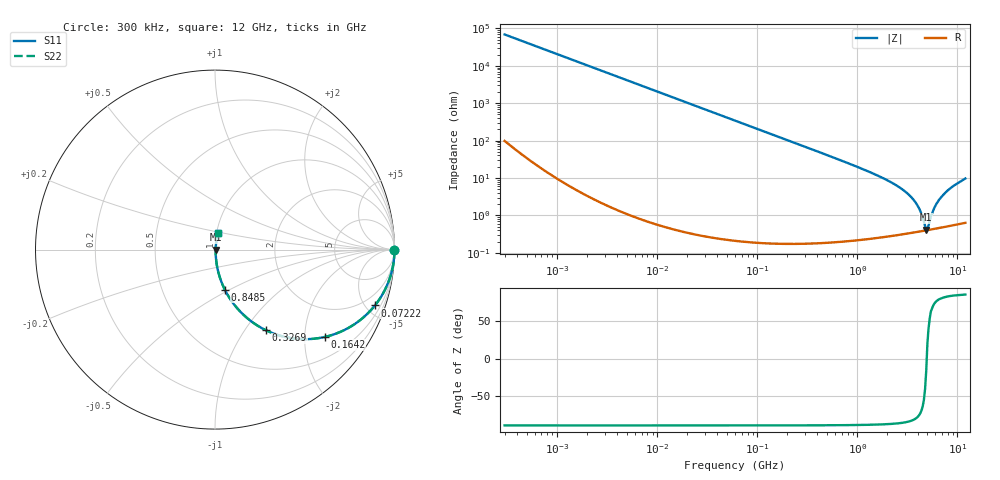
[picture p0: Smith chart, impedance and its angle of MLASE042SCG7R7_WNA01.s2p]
! MLASE042SCG7R7_WNA01  S-PARAMETER MODEL  ( General Type )
! Model Generated by TAIYO YUDEN Corporation (http://www.ty-top.com)
! Version 1.0
! TAIYO YUDEN Control No. 130801
! Copyright(c) 2013 TAIYO YUDEN CO.,LTD. All Rights Reserved.
! Product Description (link to TY-COMPAS)
! https://ds.yuden.co.jp/TYCOMPAS/or/detail?pn=MLASE042SCG7R7BWNA01&u=M
! Products Name : Multilayer Ceramic Capacitors
! Characteristics :
!  Capacitance : 7.7 pF , Rated Voltage : 16V , TCC : CG / C0G
!  Case Size : 0.4 x 0.2 / 0.016 x 0.008 [mm/inch] , Thickness : 0.2 / 0.008 [mm/inch]
!  (Conditions: Temperature = 25 degC , DC Bias Current/Voltage = 0A / 0V)
! External Node Assignments :
!  1  o---| |---o  2
! GND o---------o GND
! Frequency Range : 0.3MHz  -  12000MHz  [ 401 STEP ]
# MHz S RI R 50
! Freq[MHz].  S11 Real  S11 Imag  S21 Real  S21 Imag  S12 Real  S12 Imag  S22 Real  S22 Imag
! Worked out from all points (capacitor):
!   401 points, 300 kHz to 12 GHz, reference 50 ohm
!   read as one part in series: C = 7.7 pF near 316.3 kHz
!   lowest |Z| = 415 mohm at 4.875 GHz (marker M1)
!   series resonance near 4.934 GHz, so ESL is about 140 pH
!   S11 on the Smith chart (normalised r, x): 300 kHz: open; 72.22 MHz: 1.00, -5.72; 164.2 MHz: 1.00, -2.52; 326.9 MHz: 1.00, -1.26; 848.5 MHz: 1.00, -0.47; 12 GHz: 1.01, +0.19
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0.3  1 -0.00145  4.17e-06 0.00145  4.17e-06 0.00145  1 -0.00145
1.769972  0.9999 -0.00856  7.62e-05 0.00856  7.62e-05 0.00856  0.9999 -0.00856
10.44266  0.9974 -0.0504  0.00256 0.0504  0.00256 0.0504  0.9974 -0.0504
27.10171  0.9831 -0.1289  0.0169 0.1289  0.0169 0.1289  0.9831 -0.1289
60  0.9221 -0.2676  0.0779 0.2676  0.0779 0.2676  0.9221 -0.2676
72.22496  0.891 -0.3113  0.109 0.3113  0.109 0.3113  0.891 -0.3113
164.1901  0.6125 -0.4865  0.3875 0.4865  0.3875 0.4865  0.6125 -0.4865
326.9496  0.2844 -0.4497  0.7156 0.4497  0.7156 0.4497  0.2844 -0.4497
353.9943  0.253 -0.4332  0.747 0.4332  0.747 0.4332  0.253 -0.4332
540.8523  0.126 -0.3294  0.874 0.3294  0.874 0.3294  0.126 -0.3294
848.5281  0.0547 -0.2231  0.9453 0.2231  0.9453 0.2231  0.0547 -0.2231
2088.533  0.00926 -0.0803  0.9907 0.0803  0.9907 0.0803  0.00926 -0.0803
2870.14  0.00538 -0.0473  0.9946 0.0473  0.9946 0.0473  0.00538 -0.0473
3642.919  0.00413 -0.0257  0.9959 0.0257  0.9959 0.0257  0.00413 -0.0257
4158.869  0.00389 -0.0144  0.9961 0.0144  0.9961 0.0144  0.00389 -0.0144
4747.894  0.00392 -0.00336  0.9961 0.00336  0.9961 0.00336  0.00392 -0.00336
4875.354  0.00396 -0.00117  0.996 0.00117  0.996 0.00117  0.00396 -0.00117
5140.631  0.00407 0.00347  0.9959 -0.00347  0.9959 -0.00347  0.00407 0.00347
5868.704  0.00456 0.0151  0.9954 -0.0151  0.9954 -0.0151  0.00456 0.0151
6879.757  0.00561 0.0302  0.9944 -0.0302  0.9944 -0.0302  0.00561 0.0302
8732.115  0.00841 0.0555  0.9916 -0.0555  0.9916 -0.0555  0.00841 0.0555
12000  0.0154 0.0947  0.9846 -0.0947  0.9846 -0.0947  0.0154 0.0947
